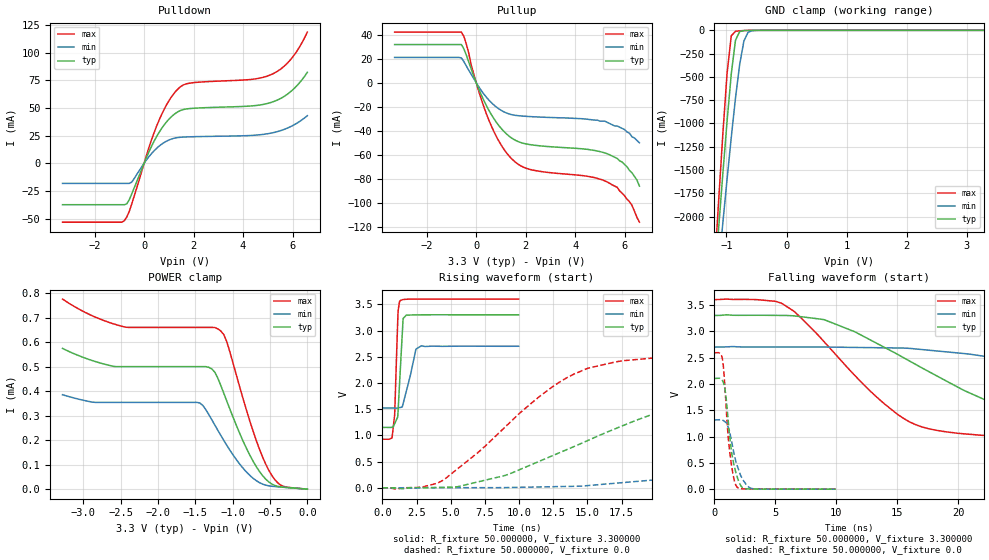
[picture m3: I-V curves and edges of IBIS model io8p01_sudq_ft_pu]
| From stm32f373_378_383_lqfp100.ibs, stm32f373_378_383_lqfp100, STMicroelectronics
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|   Model io8p01_sudq_ft_pu
[Model]  io8p01_sudq_ft_pu
Model_type I/O
Polarity   Non-Inverting
Enable   Active-Low
Vinl =   0.990000V
Vinh =   2.310000V
Vmeas =  1.650000V
Cref =   50.000000pF
Rref =   100.000000M
Vref =   0.0V
C_comp   1.970900pF   1.892300pF   2.063200pF
[Temperature Range]   25.000000   0.125000k   -40.000000
[Pullup Reference]   3.300000V   2.700000V   3.600000V
[Pulldown Reference]   0.0V   0.0V   0.0V
[POWER Clamp Reference]   3.300000V   2.700000V   3.600000V
[GND Clamp Reference]   0.0V   0.0V   0.0V
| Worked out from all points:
|   slope of the pulldown table from 0 to 0.495 V, typ, clamps not added: 20.9 ohm
|   slope of the pullup table from 0 to 0.495 V, typ, clamps not added: 22.2 ohm
|   GND clamp passes 1 mA (typ) near -0.64 V on its own axis
|   rising waveform, R_fixture 50.000000, V_fixture 3.300000: 20-80 % time 269ps typ, 640ps min, 200ps max; typ from 1.15 V to 3.3 V
|   rising waveform, R_fixture 50.000000, V_fixture 0.0: 20-80 % time 12.6ns typ, 30.5ns min, 7.07ns max; typ from 0.001 V to 2.1 V
|   falling waveform, R_fixture 50.000000, V_fixture 3.300000: 20-80 % time 10.9ns typ, 22.8ns min, 6.89ns max; typ from 3.3 V to 1.15 V
|   falling waveform, R_fixture 50.000000, V_fixture 0.0: 20-80 % time 665ps typ, 860ps min, 543ps max; typ from 2.1 V to 0.001 V
[Pulldown]
|Voltage   I(typ)   I(min)   I(max)
-3.3V     -37.45mA   -18.2mA    -53.24mA
-800mV    -37.45mA   -18.2mA    -51.9mA
-700mV    -36.7mA    -18.2mA    -48.48mA
-500mV    -27.71mA   -17.01mA   -36.65mA
500mV     23.91mA    13.38mA    33.24mA
900mV     37.17mA    19.88mA    52.48mA
1.3V      45.55mA    23.01mA    65.5mA
1.8V      49.29mA    23.83mA    72.18mA
4.4V      51.88mA    25.21mA    75.91mA
5.2V      55.41mA    27.53mA    80.72mA
5.9V      64.2mA     32.82mA    93.01mA
6.6V      82.13mA    42.97mA    118.5mA
[Pullup]
|Voltage   I(typ)   I(min)   I(max)
-3.3V     31.71mA    20.99mA    42.06mA
-600mV    31.71mA    20.58mA    42.06mA
-400mV    22.98mA    13.87mA    32.1mA
0V        90fA       16.1pA     0A
500mV     -22.5mA    -14.16mA   -30.52mA
900mV     -35.28mA   -21.55mA   -48mA
1.4V      -45.55mA   -26.41mA   -62.54mA
2.2V      -51.57mA   -28.22mA   -72.25mA
5.3V      -59.1mA    -33mA      -82.6mA
5.7V      -63mA      -36mA      -87mA
6.2V      -73mA      -42mA      -99mA
6.6V      -86mA      -50mA      -116mA
[GND_clamp]
|Voltage   I(typ)   I(min)   I(max)
-3.3V     -9.525A    -9.501A    -9.513A
-1.2V     -2.719A    -3.023A    -2.568A
-1.13V    -2.122A    -2.541A    -1.826A
-1.06V    -1.537A    -2.065A    -1.111A
-990mV    -975.7mA   -1.599A    -462mA
-920mV    -467.4mA   -1.149A    -59mA
-850mV    -106.6mA   -727.3mA   -10.11mA
-780mV    -13.06mA   -365.4mA   -5.254mA
-710mV    -3.045mA   -114.8mA   -2.635mA
-640mV    -943.2uA   -20.16mA   -905.7uA
-570mV    -199.4uA   -3.959mA   -156.8uA
3.28V     0A         0A         0A
[POWER_clamp]
|Voltage   I(typ)   I(min)   I(max)
-3.28V    574uA      385.1uA    775.2uA
-2.88V    524.3uA    354.9uA    706.9uA
-2.44V    499.6uA    353.9uA    660.7uA
-1.44V    499.6uA    351.4uA    659.6uA
-1.28V    490.1uA    283.2uA    659.6uA
-1.16V    423.2uA    219.6uA    645uA
-1.08V    359.8uA    179.3uA    602.1uA
-800mV    156.6uA    65uA       306.5uA
-640mV    71.59uA    26.48uA    162uA
-520mV    30.4uA     13.8uA     79.2uA
-360mV    9.635uA    8.674uA    17.24uA
0V        0A         0A         0A
[Ramp]
| variable   typ   min   max
dV/dt_r  1.26228/12.61797n   0.78952/30.42228n   1.55421/7.05616n
dV/dt_f  1.28868/10.87235n   0.70572/22.79880n   1.60392/6.88172n
R_load = 50.000000
[Rising Waveform]
R_fixture= 50.000000
V_fixture= 3.300000
V_fixture_min= 2.700000
V_fixture_max= 3.600000
|time   V(typ)   V(min)   V(max)
0s        1.152V     1.524V     926.8mV
720.7ps   1.154V     1.523V     980.8mV
900.9ps   1.224V     1.522V     1.396V
1.141ns   1.424V     1.525V     3.317V
1.261ns   2.003V     1.53V      3.557V
1.522ns   3.23V      1.607V     3.591V
1.762ns   3.296V     1.853V     3.596V
2.462ns   3.299V     2.646V     3.599V
2.863ns   3.3V       2.709V     3.599V
9.97ns    3.3V       2.7V       3.6V
[Rising Waveform]
R_fixture= 50.000000
V_fixture= 0.0
V_fixture_min= 0.0
V_fixture_max= 0.0
|time   V(typ)   V(min)   V(max)
0s        1.102mV    1.228mV    1.054mV
4.505ns   9.75mV     3.271mV    154.5mV
9.009ns   238.2mV    4.996mV    1.167V
14.01ns   786.9mV    29.27mV    2.169V
22.02ns   1.592V     198mV      2.526V
27.53ns   1.886V     332.4mV    2.56V
38.54ns   2.055V     659.5mV    2.588V
55.56ns   2.101V     1.056V     2.592V
75.08ns   2.104V     1.241V     2.591V
249.2ns   2.105V     1.317V     2.592V
[Falling Waveform]
R_fixture= 50.000000
V_fixture= 3.300000
V_fixture_min= 2.700000
V_fixture_max= 3.600000
|time   V(typ)   V(min)   V(max)
0s        3.3V       2.7V       3.6V
5.506ns   3.3V       2.701V     3.532V
9.009ns   3.22V      2.7V       2.799V
13.01ns   2.808V     2.688V     1.815V
16.02ns   2.435V     2.675V     1.278V
22.52ns   1.666V     2.512V     1.015V
27.53ns   1.377V     2.339V     970.5mV
41.54ns   1.204V     1.849V     936.2mV
69.57ns   1.158V     1.588V     927mV
249.2ns   1.152V     1.524V     926.8mV
[Falling Waveform]
R_fixture= 50.000000
V_fixture= 0.0
V_fixture_min= 0.0
V_fixture_max= 0.0
|time   V(typ)   V(min)   V(max)
0s        2.105V     1.317V     2.592V
660.7ps   2.063V     1.316V     2.467V
900.9ps   1.841V     1.274V     1.796V
1.141ns   1.274V     1.166V     952.7mV
1.261ns   976.7mV    1.075V     695mV
1.602ns   464.4mV    685.9mV    193.9mV
1.862ns   238mV      452mV      38.35mV
2.282ns   34.99mV    204mV      8.533mV
3.103ns   3.072mV    11.74mV    4.654mV
9.97ns    1.102mV    1.228mV    1.054mV
